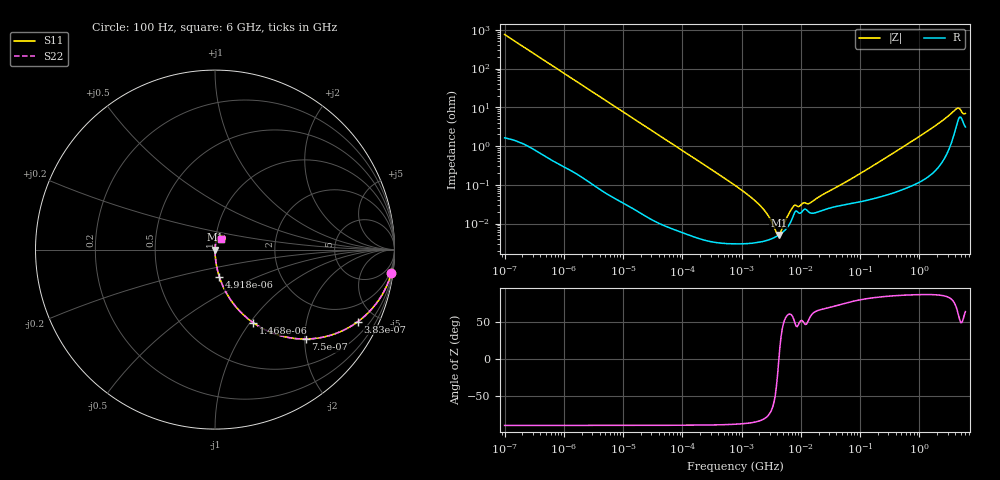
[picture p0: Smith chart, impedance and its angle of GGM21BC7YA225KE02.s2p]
!Murata Part Number: GGM21BC7YA225KE02
!These Parameters are Measured in Series Mode Connection
!Data Generated on Jun 19, 2026
!  o--ll--o
!Port1  Port2
!  o------o
!Operation Temp=25[degC], DC Bias Voltage=0[V]
!Freq. Start=100[Hz] Stop=6[GHz] 401[Steps]
# Hz S RI R 50
!Freq.(Hz) S11(Real) S11(Imag) S21(Real) S21(Imag) S12(Real) S12(Imag) S22(Real) S22(Imag)
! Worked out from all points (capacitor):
!   401 points, 100 Hz to 6 GHz, reference 50 ohm
!   read as one part in series: C = 2.1 uF near 109 Hz
!   lowest |Z| = 5.03 mohm at 4.246 MHz (marker M1)
!   series resonance near 4.266 MHz, so ESL is about 660 pH
!   S11 on the Smith chart (normalised r, x): 100 Hz: 1, -15; 383 Hz: 1.01, -3.96; 750 Hz: 1.01, -2.02; 1.468 kHz: 1.00, -1.04; 4.918 kHz: 1.00, -0.31; 6 GHz: 1.06, +0.12
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100  0.9825 -0.1299  0.0175 0.1299  0.0175 0.1299  0.9825 -0.1299
214  0.9253 -0.2614  0.0747 0.2614  0.0747 0.2614  0.9253 -0.2614
383  0.7958 -0.4014  0.2042 0.4014  0.2042 0.4014  0.7958 -0.4014
750  0.5062 -0.4982  0.4938 0.4982  0.4938 0.4982  0.5062 -0.4982
1468  0.2126 -0.4071  0.7874 0.4071  0.7874 0.4071  0.2126 -0.4071
2008  0.1267 -0.3305  0.8733 0.3305  0.8733 0.3305  0.1267 -0.3305
4918  0.0241 -0.1513  0.9759 0.1513  0.9759 0.1513  0.0241 -0.1513
12041  0.0043 -0.0632  0.9957 0.0632  0.9957 0.0632  0.0043 -0.0632
40335  0.000462 -0.019  0.9995 0.019  0.9995 0.019  0.000462 -0.019
774597  3.07e-05 -0.000964  1 0.000964  1 0.000964  3.07e-05 -0.000964
1896632  3.26e-05 -0.000327  1 0.000327  1 0.000327  3.26e-05 -0.000327
2481164  3.55e-05 -0.000207  1 0.000207  1 0.000207  3.55e-05 -0.000207
3394479  4.19e-05 -8.44e-05  1 8.44e-05  1 8.44e-05  4.19e-05 -8.44e-05
4246196  5.03e-05 -1.7e-06  0.9999 1.7e-06  0.9999 1.7e-06  5.03e-05 -1.7e-06
5311619  6.56e-05 8.37e-05  0.9999 -8.37e-05  0.9999 -8.37e-05  6.56e-05 8.37e-05
7599586  0.000171 0.000227  0.9998 -0.000227  0.9998 -0.000227  0.000171 0.000227
1.555665e7  0.000184 0.000319  0.9998 -0.000319  0.9998 -0.000319  0.000184 0.000319
3.124326e8  0.000601 0.00564  0.9994 -0.00564  0.9994 -0.00564  0.000601 0.00564
1.712697e9  0.00295 0.0303  0.9971 -0.0303  0.9971 -0.0303  0.00295 0.0303
4.193612e9  0.0371 0.0792  0.9629 -0.0792  0.9629 -0.0792  0.0371 0.0792
4.586474e9  0.0531 0.0737  0.9469 -0.0737  0.9469 -0.0737  0.0531 0.0737
6e9  0.0336 0.0581  0.9664 -0.0581  0.9664 -0.0581  0.0336 0.0581
